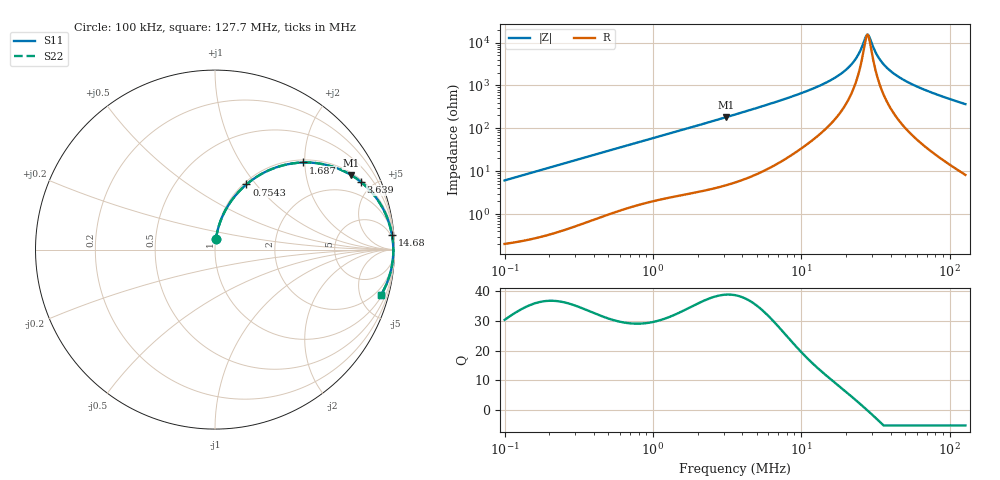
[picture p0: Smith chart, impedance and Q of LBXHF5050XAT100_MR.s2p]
! LBXHF5050XAT100_MR  S-PARAMETER MODEL  ( General Type )
! Model Generated by TAIYO YUDEN Corporation (http://www.ty-top.com)
! Version 1.0
! TAIYO YUDEN Control No. 201105NI43SB-FBB
! Copyright(c) 2020 TAIYO YUDEN CO.,LTD. All Rights Reserved.
! Product Description (link to TY-COMPAS)
! https://ds.yuden.co.jp/TYCOMPAS/or/detail?pn=LBXHF5050XAT100MMR&u=M
! Products Name : Inductors
! Characteristics :
!  Inductance : 10 uH , SRF(min) : 20 MHz , DC Resistance(max) : 0.115 Ohm
!  Rated Current : Saturation :2500 mA , Temp Rise : 1100 mA
!  Case Size : 5.0 x 5.0 / 0.197 x 0.197 [mm/inch] , Thickness : 3.1 / 0.122 [mm/inch]
!  (Conditions: Temperature = 25 degC , DC Bias Current/Voltage = 0A / 0V)
! External Node Assignments :
!  1  o---GGG---o  2
! GND o---------o GND
! Frequency Range : 0.1MHz  -  127.746476MHz  [ 402 STEP ]
# MHz S RI R 50
! Freq[MHz].  S11 Real  S11 Imag  S21 Real  S21 Imag  S12 Real  S12 Imag  S22 Real  S22 Imag
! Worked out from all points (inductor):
!   401 points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, 100 kHz to 127.7 MHz, reference 50 ohm
!   read as one part in series: L = 9.68 uH near 103.6 kHz
!   highest Q = 38.6 at 3.098 MHz (marker M1), where L = 9.3 uH
!   self-resonance near 27.94 MHz
!   S11 on the Smith chart (normalised r, x): 100 kHz: 1.00, +0.12; 754.3 kHz: 1.03, +0.89; 1.687 MHz: 1.06, +1.97; 3.639 MHz: 1.11, +4.27; 14.68 MHz: 3, +23; 127.7 MHz: 1.16, -7.33
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0.1  0.00569 0.0605  0.9943 -0.0605  0.9943 -0.0605  0.00569 0.0605
0.33137  0.0436 0.1901  0.9564 -0.1901  0.9564 -0.1901  0.0436 0.1901
0.754299  0.175 0.3631  0.825 -0.3631  0.825 -0.3631  0.175 0.3631
1.098062  0.2997 0.4418  0.7003 -0.4418  0.7003 -0.4418  0.2997 0.4418
1.686583  0.4918 0.4854  0.5082 -0.4854  0.5082 -0.4854  0.4918 0.4854
3.097758  0.7605 0.4141  0.2395 -0.4141  0.2395 -0.4141  0.7605 0.4141
3.574164  0.8083 0.3808  0.1917 -0.3808  0.1917 -0.3808  0.8083 0.3808
3.63865  0.8138 0.3765  0.1862 -0.3765  0.1862 -0.3765  0.8138 0.3765
6.11154  0.925 0.2478  0.075 -0.2478  0.075 -0.2478  0.925 0.2478
11.84371  0.9785 0.1168  0.0215 -0.1168  0.0215 -0.1168  0.9785 0.1168
14.67839  0.9856 0.084  0.0144 -0.084  0.0144 -0.084  0.9856 0.084
18.51973  0.9903 0.052  0.00965 -0.052  0.00965 -0.052  0.9903 0.052
21.75342  0.9923 0.0313  0.00768 -0.0313  0.00768 -0.0313  0.9923 0.0313
24.21714  0.9931 0.0178  0.00689 -0.0178  0.00689 -0.0178  0.9931 0.0178
26.95988  0.9935 0.00453  0.00649 -0.00453  0.00649 -0.00453  0.9935 0.00453
27.9415  0.9936 0.000119  0.00643 -0.000119  0.00643 -0.000119  0.9936 0.000119
28.95886  0.9936 -0.0043  0.00642 0.0043  0.00642 0.0043  0.9936 -0.0043
33.41246  0.9932 -0.0221  0.00679 0.0221  0.00679 0.0221  0.9932 -0.0221
39.24654  0.992 -0.0426  0.00804 0.0426  0.00804 0.0426  0.992 -0.0426
47.77778  0.989 -0.0691  0.011 0.0691  0.011 0.0691  0.989 -0.0691
61.36888  0.9824 -0.1064  0.0176 0.1064  0.0176 0.1064  0.9824 -0.1064
127.7465  0.926 -0.2508  0.074 0.2508  0.074 0.2508  0.926 -0.2508
